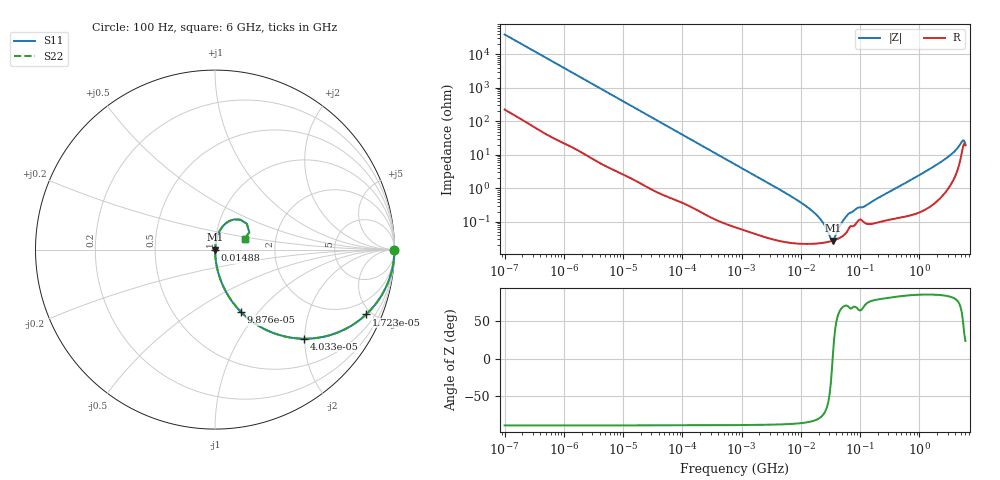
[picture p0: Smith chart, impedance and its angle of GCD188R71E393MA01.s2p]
!Murata Part Number: GCD188R71E393MA01
!These Parameters are Measured in Series Mode Connection
!Data Generated on Jan 08, 2026
!  o--ll--o
!Port1  Port2
!  o------o
!Operation Temp=25[degC], DC Bias Voltage=0[V]
!Freq. Start=100[Hz] Stop=6[GHz] 401[Steps]
# Hz S RI R 50
!Freq.(Hz) S11(Real) S11(Imag) S21(Real) S21(Imag) S12(Real) S12(Imag) S22(Real) S22(Imag)
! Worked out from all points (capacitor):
!   401 points, 100 Hz to 6 GHz, reference 50 ohm
!   read as one part in series: C = 40.4 nF near 109 Hz
!   lowest |Z| = 27.9 mohm at 34.83 MHz (marker M1)
!   series resonance near 34.48 MHz, so ESL is about 530 pH
!   S11 on the Smith chart (normalised r, x): 100 Hz: open; 17.23 kHz: 1.03, -4.65; 40.34 kHz: 1.01, -1.99; 98.76 kHz: 1.01, -0.82; 14.88 MHz: 1.00, -0.00; 6 GHz: 1.38, +0.17
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100  1 -0.00254  2.11e-05 0.00254  2.11e-05 0.00254  1 -0.00254
2008  0.9972 -0.0504  0.00285 0.0504  0.00285 0.0504  0.9972 -0.0504
7695  0.9631 -0.1854  0.0369 0.1854  0.0369 0.1854  0.9631 -0.1854
17227  0.8422 -0.3611  0.1578 0.3611  0.1578 0.3611  0.8422 -0.3611
40335  0.4983 -0.4964  0.5017 0.4964  0.5017 0.4964  0.4983 -0.4964
98762  0.1455 -0.348  0.8545 0.348  0.8545 0.348  0.1455 -0.348
264476  0.0245 -0.1496  0.9755 0.1496  0.9755 0.1496  0.0245 -0.1496
774597  0.00346 -0.0525  0.9965 0.0525  0.9965 0.0525  0.00346 -0.0525
6075234  0.000286 -0.0066  0.9997 0.0066  0.9997 0.0066  0.000286 -0.0066
1.487547e7  0.000227 -0.00227  0.9998 0.00227  0.9998 0.00227  0.000227 -0.00227
1.555665e7  0.000227 -0.00212  0.9998 0.00212  0.9998 0.00212  0.000227 -0.00212
2.225763e7  0.000236 -0.00109  0.9998 0.00109  0.9998 0.00109  0.000236 -0.00109
3.184506e7  0.000265 -0.000192  0.9997 0.000192  0.9997 0.000192  0.000265 -0.000192
3.482834e7  0.000277 2.46e-05  0.9997 -2.46e-05  0.9997 -2.46e-05  0.000277 2.46e-05
4.983056e7  0.00037 0.000925  0.9996 -0.000925  0.9996 -0.000925  0.00037 0.000925
6.518806e7  0.000654 0.00168  0.9993 -0.00168  0.9993 -0.00168  0.000654 0.00168
3.124326e8  0.00122 0.00785  0.9988 -0.00785  0.9988 -0.00785  0.00122 0.00785
1.497423e9  0.00421 0.0377  0.9958 -0.0377  0.9958 -0.0377  0.00421 0.0377
3.352442e9  0.0215 0.0952  0.9785 -0.0952  0.9785 -0.0952  0.0215 0.0952
4.385646e9  0.0539 0.1409  0.9461 -0.1409  0.9461 -0.1409  0.0539 0.1409
5.245841e9  0.141 0.1667  0.859 -0.1667  0.859 -0.1667  0.141 0.1667
6e9  0.1655 0.0588  0.8345 -0.0588  0.8345 -0.0588  0.1655 0.0588
